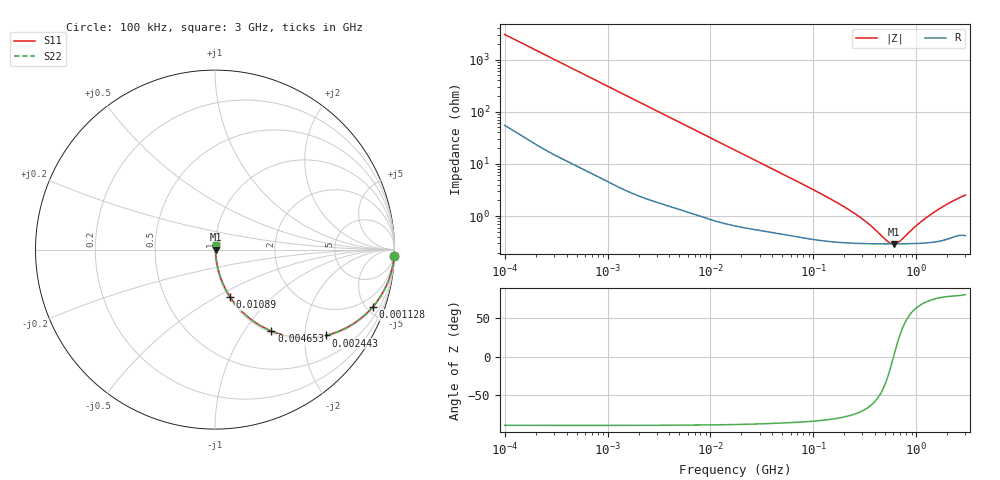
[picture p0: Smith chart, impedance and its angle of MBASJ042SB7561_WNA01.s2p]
! MBASJ042SB7561_WNA01  S-PARAMETER MODEL  ( Standard Model )
! Model Generated by TAIYO YUDEN Corporation (https://www.yuden.co.jp/en/)
! Version 1.0
! TAIYO YUDEN Control No. 250312
! Copyright(c) 2025 TAIYO YUDEN CO.,LTD. All Rights Reserved.
! Product Description (link to TY-COMPAS)
! https://ds.yuden.co.jp/TYCOMPAS/or/detail?pn=MBASJ042SB7561KWNA01&u=M
! Products Name : Multilayer Ceramic Capacitors
! Characteristics :
!  Capacitance : 560 [pF] , Rated Voltage : 6.3 [V] , TCC : X7R
!  Case Size : 0.4 x 0.2 / 0.016 x 0.008 [mm/inch] , Thickness : 0.2 / 0.008 [mm/inch]
!  (Conditions: Temperature = 25 [degC] , DC Bias Voltage = 0 [V])
! External Node Assignments :
!  1  o---| |---o  2
! GND o---------o GND
! Frequency Range : 100kHz  -  3GHz  [ 401 STEP ]
# MHZ S RI R 50
! Freq[MHz].  S11 Real  S11 Imag  S21 Real  S21 Imag  S12 Real  S12 Imag  S22 Real  S22 Imag
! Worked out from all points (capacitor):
!   401 points, 100 kHz to 3 GHz, reference 50 ohm
!   read as one part in series: C = 525 pF near 105.3 kHz
!   lowest |Z| = 293 mohm at 607 MHz (marker M1)
!   series resonance near 601.8 MHz, so ESL is about 130 pH
!   S11 on the Smith chart (normalised r, x): 100 kHz: 2, -60; 1.128 MHz: 1.08, -5.48; 2.443 MHz: 1.04, -2.54; 4.653 MHz: 1.03, -1.34; 10.89 MHz: 1.02, -0.58; 3 GHz: 1.01, +0.05
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0.1  0.9983 -0.033  0.00169 0.033  0.00169 0.033  0.9983 -0.033
0.259498  0.9916 -0.0842  0.00843 0.0842  0.00843 0.0842  0.9916 -0.0842
0.562235  0.9651 -0.1762  0.0349 0.1762  0.0349 0.1762  0.9651 -0.1762
1.127518  0.8789 -0.319  0.1211 0.319  0.1211 0.319  0.8789 -0.319
1.659646  0.7736 -0.411  0.2264 0.411  0.2264 0.411  0.7736 -0.411
2.442911  0.6161 -0.4781  0.3839 0.4781  0.3839 0.4781  0.6161 -0.4781
3.161081  0.4925 -0.491  0.5075 0.491  0.5075 0.491  0.4925 -0.491
4.652942  0.3145 -0.454  0.6855 0.454  0.6855 0.454  0.3145 -0.454
7.027689  0.1723 -0.3658  0.8277 0.3658  0.8277 0.3658  0.1723 -0.3658
10.89156  0.0837 -0.2632  0.9163 0.2632  0.9163 0.2632  0.0837 -0.2632
17.7727  0.0366 -0.1707  0.9634 0.1707  0.9634 0.1707  0.0366 -0.1707
37.52708  0.012 -0.0837  0.988 0.0837  0.988 0.0837  0.012 -0.0837
97.38194  0.00463 -0.0325  0.9954 0.0325  0.9954 0.0325  0.00463 -0.0325
266.0711  0.00309 -0.00993  0.9969 0.00993  0.9969 0.00993  0.00309 -0.00993
353.2796  0.00298 -0.0061  0.997 0.0061  0.997 0.0061  0.00298 -0.0061
547.5153  0.00292 -0.00103  0.9971 0.00103  0.9971 0.00103  0.00292 -0.00103
606.9703  0.00292 9.54e-05  0.9971 -9.54e-05  0.9971 -9.54e-05  0.00292 9.54e-05
690.4488  0.00293 0.00151  0.9971 -0.00151  0.9971 -0.00151  0.00293 0.00151
1042.837  0.00303 0.00634  0.997 -0.00634  0.997 -0.00634  0.00303 0.00634
1457.883  0.00327 0.011  0.9967 -0.011  0.9967 -0.011  0.00327 0.011
2145.926  0.00409 0.0179  0.9959 -0.0179  0.9959 -0.0179  0.00409 0.0179
3000  0.00484 0.0248  0.9952 -0.0248  0.9952 -0.0248  0.00484 0.0248
